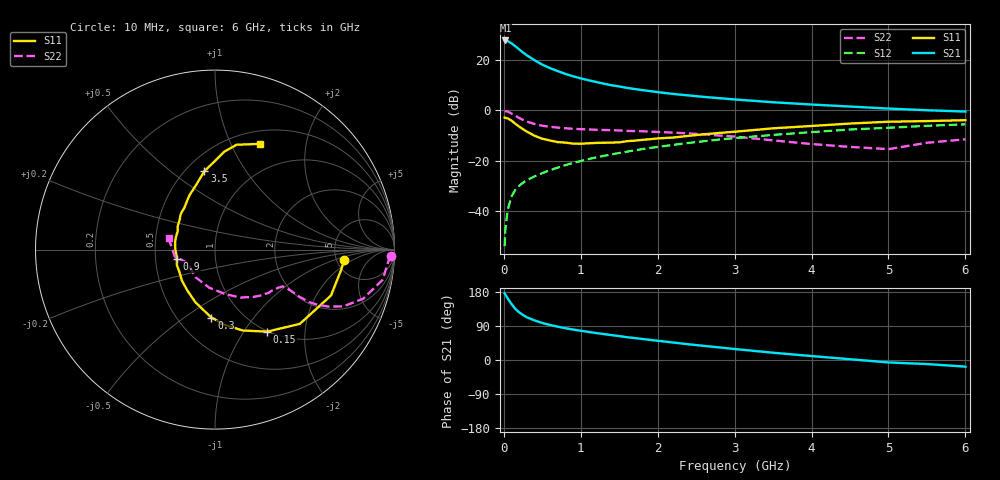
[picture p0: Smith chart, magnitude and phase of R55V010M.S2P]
! SIEMENS Small Signal Semiconductors
! BFR183
! Si NPN RF Bipolar Junction Transistor in SOT23
! VCE = 5 V  IC = 10 mA
! Common Emitter S-Parameters:  May  1996
# GHz  S  MA  R  50
!  f  S11  S21  S12  S22
! GHz  MAG  ANG  MAG  ANG  MAG  ANG  MAG  ANG
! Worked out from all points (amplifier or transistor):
!   36 points, 10 MHz to 6 GHz, reference 50 ohm
!   highest |S21| = 27.8 dB at 20 MHz (marker M1)
!   |S21| within 3 dB of that: start of sweep to 177.2 MHz
!   unconditionally stable (mu >= 1): 801.1 MHz to 2.524 GHz
!   at 250 MHz: K = 0.62, MSG = 25.9 dB, |S12| = -28.7 dB
!   at 1.4 GHz: K = 1.05, MAG = 12.3 dB, |S12| = -17.5 dB
!   at 6 GHz: K = 0.89, MSG = 2.5 dB, |S12| = -5.5 dB
!   lowest NFmin = 1.30 dB at 450 MHz
!   S11 on the Smith chart (normalised r, x): 10 MHz: 5.85, -1.38; 150 MHz: 0.99, -1.28; 300 MHz: 0.72, -0.64; 900 MHz: 0.65, -0.07; 3.5 GHz: 0.61, +0.67; 6 GHz: 0.65, +1.30
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0.01  0.7216 -4.5  24.56 176.3  0.002 85.0  0.9785 -2.0
0.02  0.7122 -9.1  24.66 172.5  0.0043 86.5  0.9673 -4.1
0.05  0.6951 -21.6  24.02 162.5  0.0106 80.4  0.9491 -10.2
0.1  0.6283 -41.2  21.58 147.7  0.0195 72.4  0.8699 -18.3
0.15  0.5413 -57.6  18.86 134.7  0.0265 66.9  0.7829 -23.8
0.2  0.4764 -71.1  16.37 125.7  0.0318 64.4  0.7068 -26.7
0.25  0.4234 -82.5  14.16 118.5  0.0366 62.8  0.6477 -28.3
0.3  0.3791 -93.1  12.45 112.6  0.041 63.0  0.6025 -29.1
0.4  0.3132 -110.4  9.96 104.4  0.049 62.9  0.5364 -29.2
0.5  0.274 -124.5  8.154 97.7  0.0567 64.1  0.496 -28.7
0.6  0.2529 -136.7  6.943 92.5  0.065 64.3  0.4732 -28.4
0.7  0.2348 -147.3  6.055 87.9  0.0729 65.0  0.4561 -28.3
0.9  0.2192 -166.6  4.781 80.4  0.0907 65.8  0.4315 -28.5
1.1  0.2223 177.5  3.989 74.1  0.1076 65.4  0.4188 -30.1
1.3  0.2281 163.9  3.401 68.4  0.1253 64.6  0.4083 -31.7
1.6  0.2451 148.1  2.813 60.2  0.1517 62.9  0.393 -35.3
2.2  0.289 126.2  2.13 46.1  0.2068 58.3  0.3632 -44.6
2.8  0.3569 109.8  1.755 33.2  0.2637 52.1  0.3176 -56.6
3.5  0.4412 97.7  1.455 19.2  0.3262 43.7  0.2538 -77.1
4.5  0.5489 84.5  1.196 2.0  0.4179 31.6  0.1883 -125.1
5.5  0.6149 72.5  1.01 -10.7  0.4947 19.8  0.2275 -170.3
6  0.6403 67.0  0.95 -17.5  0.5307 12.2  0.2671 165.9
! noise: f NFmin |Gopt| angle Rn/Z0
0.45  1.3  0.15  45  0.18
0.9  1.4  0.2  125  0.19
1.8  2.1  0.34  -170  0.14
